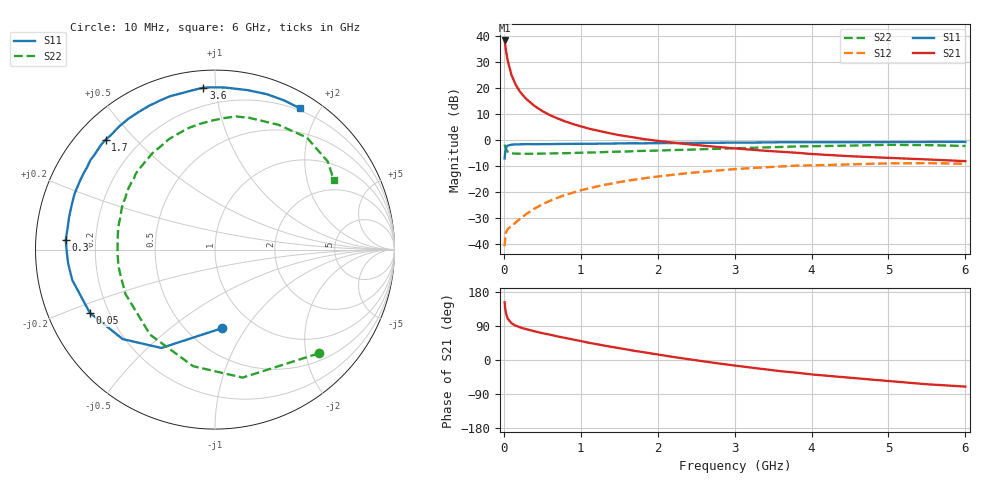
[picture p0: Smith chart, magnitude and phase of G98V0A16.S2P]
! SIEMENS Small Signal Semiconductors
! BFG235
! Si NPN RF Bipolar Junction Transistor in SOT223
! VCE = 8 V  IC = 160 mA
! Common Emitter S-Parameters:  July  1994
# GHz  S  MA  R  50
!  f  S11  S21  S12  S22
! GHz  MAG  ANG  MAG  ANG  MAG  ANG  MAG  ANG
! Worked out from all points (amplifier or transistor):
!   40 points, 10 MHz to 6 GHz, reference 50 ohm
!   highest |S21| = 38.3 dB at 10 MHz (marker M1)
!   |S21| within 3 dB of that: start of sweep to 24.27 MHz
!   unconditionally stable (mu >= 1): 460.7 MHz to 1.486 GHz
!   at 200 MHz: K = 0.81, MSG = 24.8 dB, |S12| = -30.5 dB
!   at 1.5 GHz: K = 1.00, MSG = 9.0 dB, |S12| = -16.2 dB
!   at 6 GHz: K = 0.89, MSG = 0.5 dB, |S12| = -9.1 dB
!   S11 on the Smith chart (normalised r, x): 10 MHz: 0.72, -0.78; 50 MHz: 0.13, -0.23; 300 MHz: 0.09, +0.03; 1.7 GHz: 0.09, +0.41; 3.6 GHz: 0.09, +0.93; 6 GHz: 0.17, +1.75
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0.01  0.4401 -85.2  81.82 152.3  0.0091 63.7  0.8176 -45.0
0.02  0.6243 -118.6  64.24 133.4  0.0143 48.9  0.7297 -77.8
0.03  0.7164 -135.9  50.41 121.6  0.017 40.1  0.6609 -100.6
0.05  0.7813 -153.2  33.55 109.0  0.0193 33.8  0.5962 -127.3
0.1  0.8133 -168.0  17.69 97.0  0.0225 36.2  0.5568 -153.7
0.15  0.8221 -174.8  11.9 90.9  0.0256 43.1  0.5456 -164.6
0.2  0.8251 -178.4  8.892 87.0  0.0297 47.5  0.5454 -170.8
0.25  0.8293 178.5  7.166 83.6  0.034 51.6  0.5432 -175.1
0.3  0.8339 176.3  5.986 81.0  0.0384 53.7  0.5431 -178.7
0.4  0.8296 171.7  4.501 75.6  0.0481 56.9  0.5436 176.3
0.5  0.8326 167.9  3.596 70.9  0.0579 58.0  0.547 172.1
0.6  0.834 164.8  2.999 66.8  0.0678 58.1  0.5512 168.2
0.8  0.8417 158.5  2.263 58.2  0.0881 56.4  0.5568 161.5
1.1  0.8467 149.5  1.661 45.6  0.1172 51.7  0.5742 152.5
1.4  0.8542 142.2  1.326 34.7  0.1451 45.8  0.5917 144.3
1.7  0.8639 134.8  1.113 24.1  0.1731 39.5  0.6104 136.5
2.2  0.8742 123.6  0.889 8.1  0.2148 28.5  0.6406 122.9
3.2  0.8909 102.2  0.653 -19.7  0.2874 5.4  0.7048 97.1
3.6  0.9048 94.1  0.594 -29.6  0.3098 -4.5  0.7344 86.1
4.5  0.9071 78.3  0.488 -46.8  0.3396 -24.3  0.7797 63.2
5.5  0.9161 65.0  0.423 -64.0  0.3592 -46.3  0.7972 38.0
6  0.9182 59.0  0.392 -70.2  0.3493 -54.6  0.7674 30.5
